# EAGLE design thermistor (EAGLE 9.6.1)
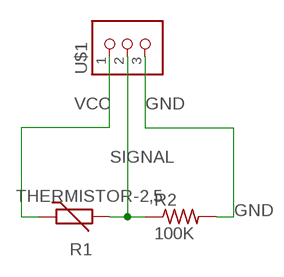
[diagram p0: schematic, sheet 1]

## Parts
R1  THERMISTOR-2,5  [RS-2,5]
R2  100K  RES-US1206FAB  [R1206FAB]
U$1  TERM-1X03'-FABLAB'  [ED555DS-3DS]

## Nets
GND: R2.2 U$1.3
SIGNAL: R1.2 R2.1 U$1.2
VCC: R1.1 U$1.1

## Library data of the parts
R1 = varistor:THERMISTOR: THERMISTOR
R2 = fab:RES-US: Resistor (US Symbol)
U$1 = fab:TERM-1X03: 3.5mm terminal block, 3 positions ED555-3DS as found in the fablab inventory. Made by Zaerc.

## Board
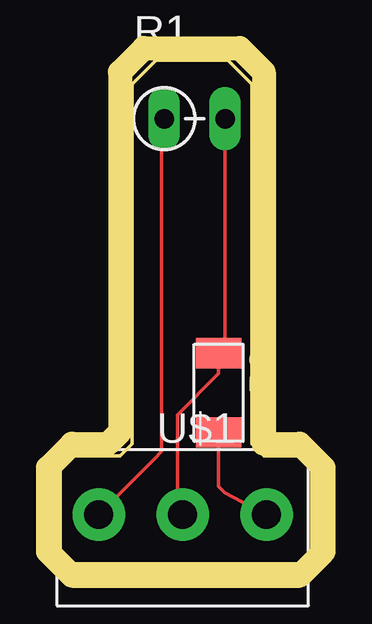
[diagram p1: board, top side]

Size 10.5 x 21 mm. Coordinates in mm from the lower left corner, seen from the top.
Outline: 10.5,4 10,4.5 8.5,4.5 8,5 8,20 7,21 4,21 3,20 3,5 2.5,4.5 0.5,4.5 0,4 0,0.5 0.5,0 10,0 10.5,0.5 10.5,4
Copper layers (1*16): Top 0.035mm / dielectric 1.5mm / Bottom 0.035mm
Design rules "default": minimum track width 6mil, minimum drill 0.35mm, track to track 6mil, track to pad 6mil, pad to pad 6mil, via to via 6mil, smd to smd 6mil, copper to edge 40mil, drill to drill 6mil, minimum pad ring 10mil, minimum via ring 8mil, stop-mask expansion 4mil, vias tented up to drill 0mil, thermal gap 10mil
Milling: 15 lines

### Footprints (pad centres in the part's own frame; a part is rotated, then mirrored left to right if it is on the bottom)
RS-2,5 = drill 0.813 long: 1 -1.27,0; 2 1.27,0
R1206FAB = smd 1.27 x 1.905: 1 -1.651,0; 2 1.651,0
ED555DS-3DS = drill 1.2 pad 2.184: 1 -3.5,0; 2 0,0; 3 3.5,0

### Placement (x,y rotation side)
R1  5.62,18.55 0 top
R2  6.62,7.12 270 top
U$1  5.12,2.04 0 top

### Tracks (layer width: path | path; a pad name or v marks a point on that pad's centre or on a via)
GND
  Top 0.152: R2.2 6.62,3.22 6.9,2.95 U$1.3
SIGNAL
  Top 0.152: 6.62,8.5 6.62,7.93 4.9,6.21 4.9,2.26 U$1.2 | 6.62,8.5 R2.1 | R1.2 6.89,8.77 6.62,8.5
VCC
  Top 0.152: R1.1 4.25,18.55 4.25,4.68 3.93,4.35 U$1.1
